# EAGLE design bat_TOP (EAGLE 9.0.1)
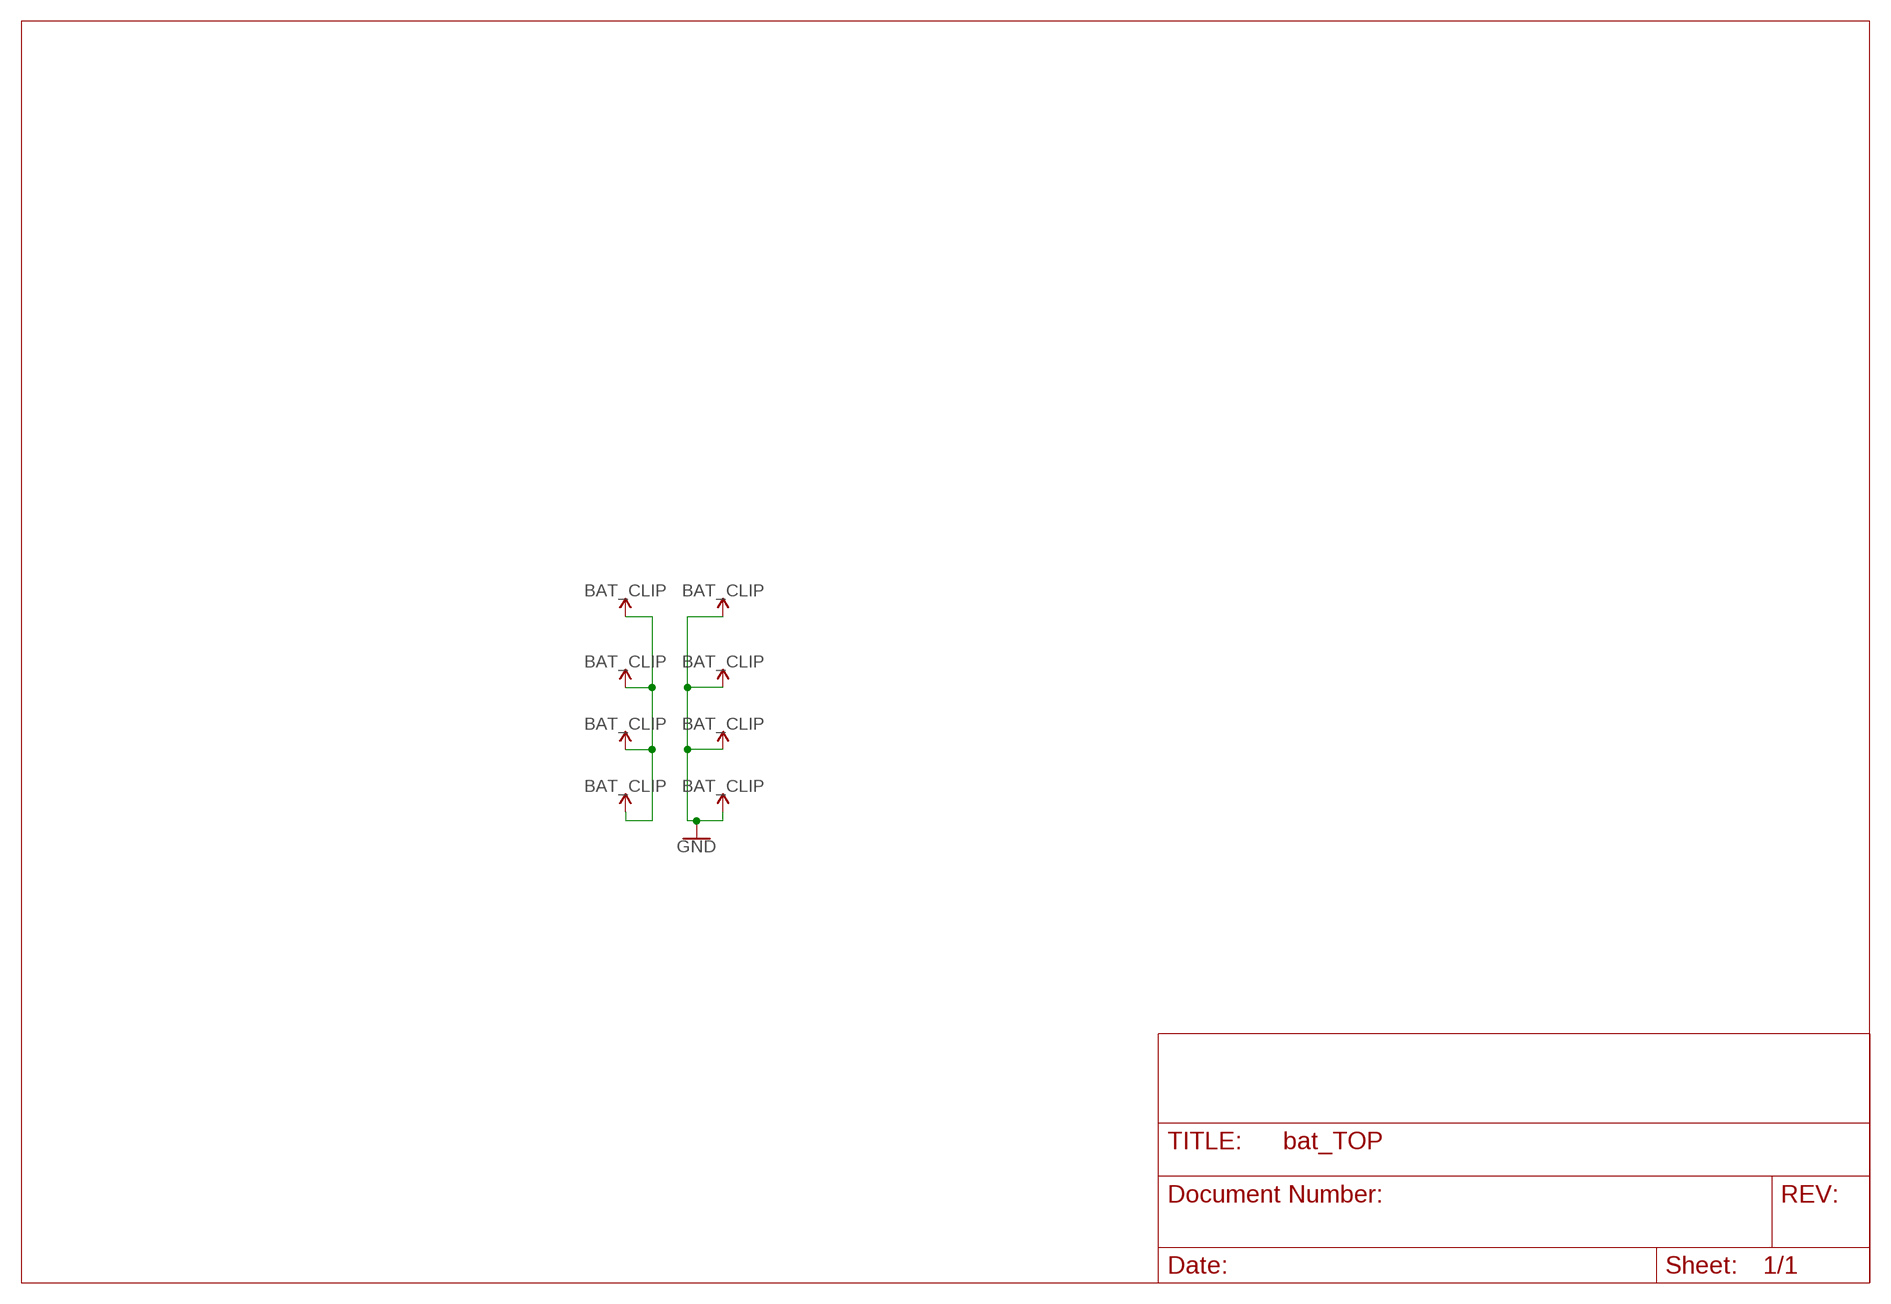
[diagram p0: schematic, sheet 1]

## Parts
U$1  BAT_CLIP  [CLIP]
U$2  BAT_CLIP  [CLIP]
U$3  BAT_CLIP  [CLIP]
U$4  BAT_CLIP  [CLIP]
U$5  BAT_CLIP  [CLIP]
U$6  BAT_CLIP  [CLIP]
U$7  BAT_CLIP  [CLIP]
U$8  BAT_CLIP  [CLIP]

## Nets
GND: U$2.P$1(V_BATT) U$2.P$2(V_BATT) U$2.P$3(V_BATT) U$2.P$4(V_BATT) U$5.P$1(V_BATT) U$5.P$2(V_BATT) U$5.P$3(V_BATT) U$5.P$4(V_BATT) U$6.P$1(V_BATT) U$6.P$2(V_BATT) U$6.P$3(V_BATT) U$6.P$4(V_BATT) U$8.P$1(V_BATT) U$8.P$2(V_BATT) U$8.P$3(V_BATT) U$8.P$4(V_BATT)
V_BATT: U$1.P$1(V_BATT) U$1.P$2(V_BATT) U$1.P$3(V_BATT) U$1.P$4(V_BATT) U$3.P$1(V_BATT) U$3.P$2(V_BATT) U$3.P$3(V_BATT) U$3.P$4(V_BATT) U$4.P$1(V_BATT) U$4.P$2(V_BATT) U$4.P$3(V_BATT) U$4.P$4(V_BATT) U$7.P$1(V_BATT) U$7.P$2(V_BATT) U$7.P$3(V_BATT) U$7.P$4(V_BATT)

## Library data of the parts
U$1-U$8 = bat:BAT_CLIP

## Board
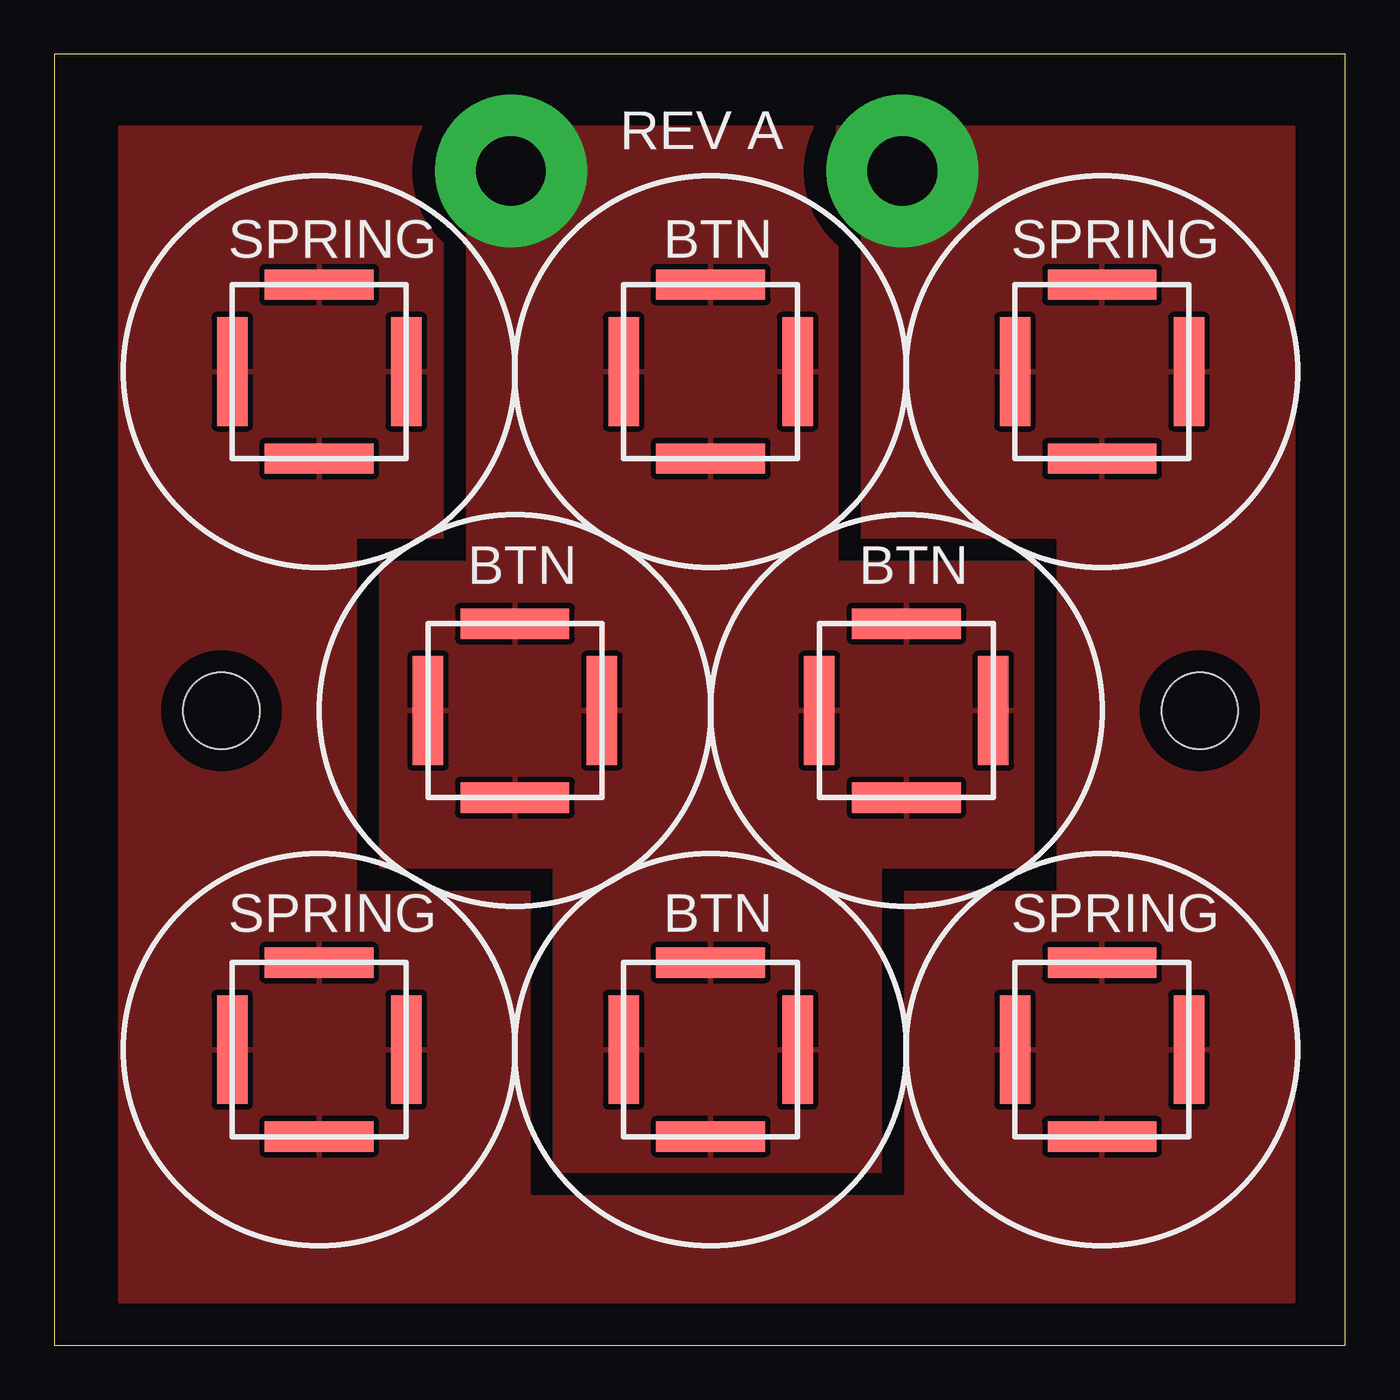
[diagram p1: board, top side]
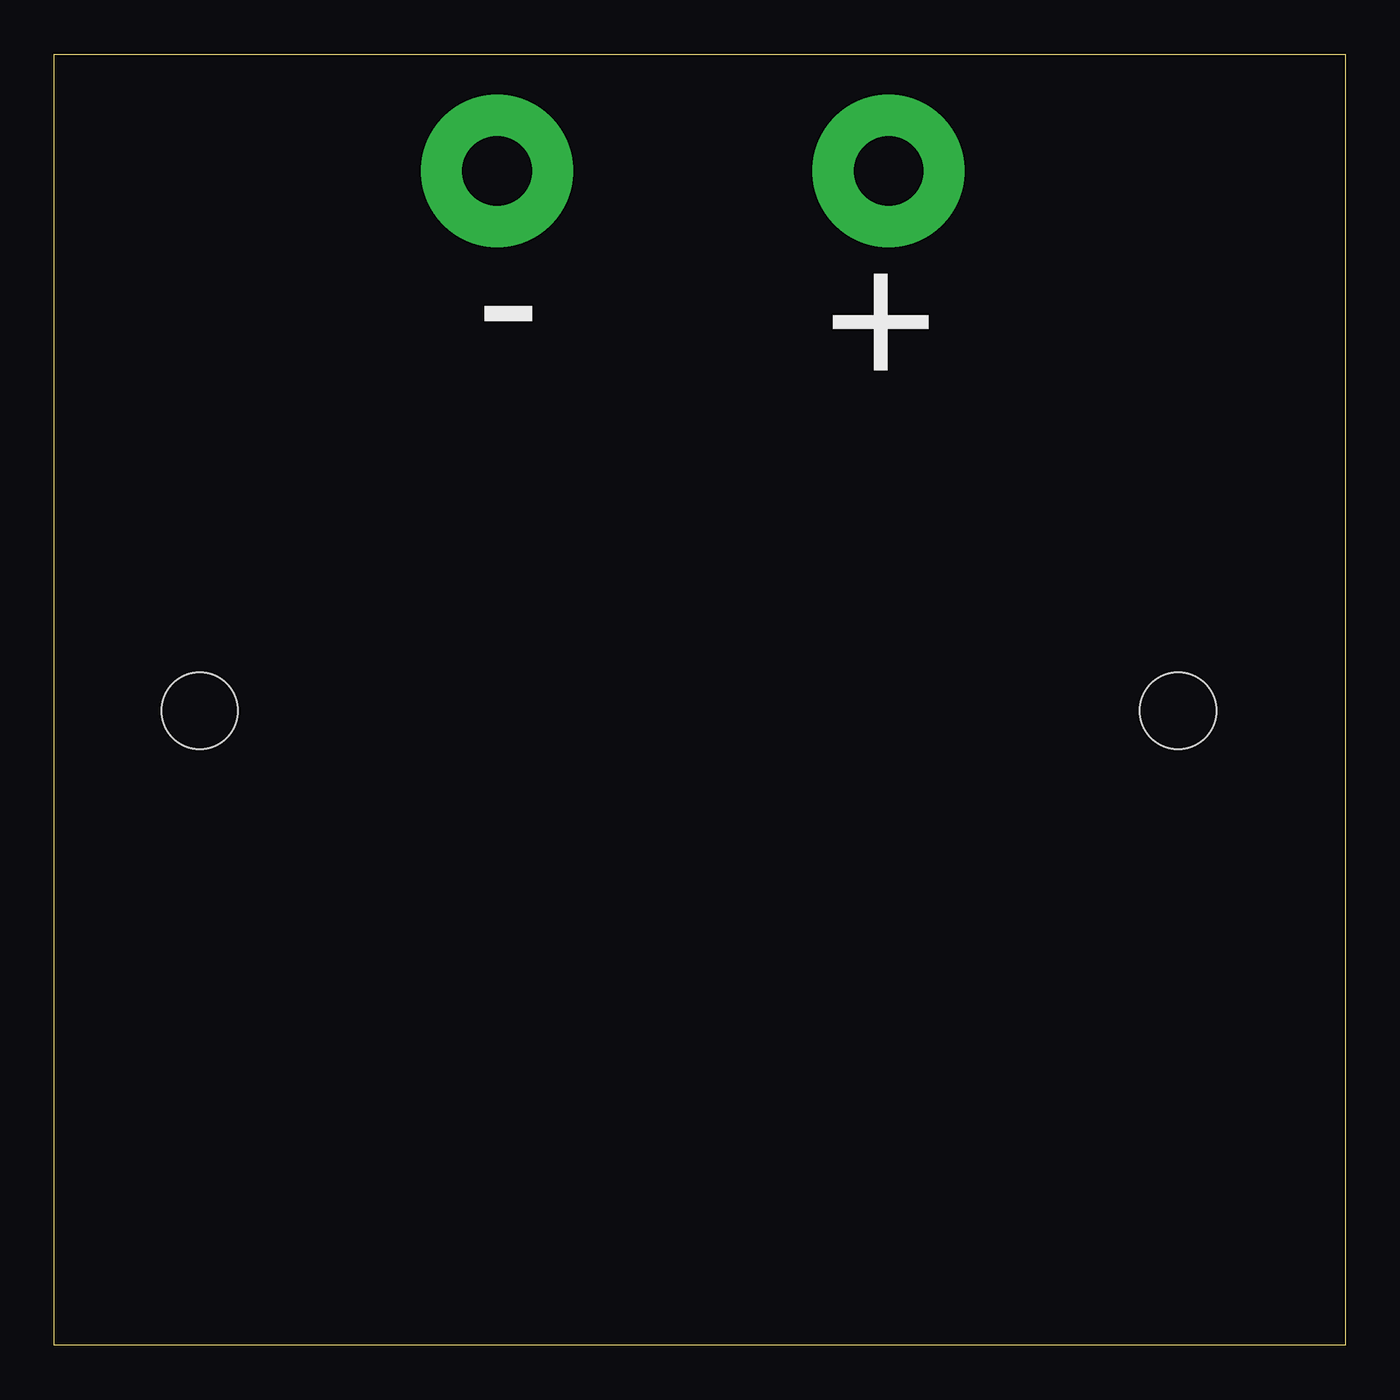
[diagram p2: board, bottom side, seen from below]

Size 59.36 x 59.36 mm. Coordinates in mm from the lower left corner, seen from the top.
Outline: 0,0 59.36,0 59.36,59.36 0,59.36 0,0
Copper layers (1*16): Top 0.035mm / dielectric 1.5mm / Bottom 0.035mm
Design rules "default": minimum track width 6mil, minimum drill 0.35mm, track to track 6mil, track to pad 6mil, pad to pad 6mil, via to via 6mil, smd to smd 6mil, copper to edge 40mil, drill to drill 6mil, minimum pad ring 10mil, minimum via ring 8mil, stop-mask expansion 4mil, vias tented up to drill 0mil, thermal gap 10mil
Holes 3.5 mm at 7.68,29.18 52.68,29.18

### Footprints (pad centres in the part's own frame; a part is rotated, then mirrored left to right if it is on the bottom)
CLIP = smd 1.4 x 5: P$1 -4,0; P$2 4,0 | smd 5 x 1.4: P$3 0,4; P$4 0,-4

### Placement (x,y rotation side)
U$1  21.18,29.18 0 top
U$2  12.18,13.59 0 top
U$3  39.18,29.18 0 top
U$4  30.18,13.59 0 top
U$5  12.18,44.77 0 top
U$6  48.18,44.77 0 top
U$7  30.18,44.77 0 top
U$8  48.18,13.59 0 top

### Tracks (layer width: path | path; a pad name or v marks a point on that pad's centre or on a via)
GND  (via drill 3.2 pad 7)
  other vias: 39,54
  pour Top (isolate 1.016, rank 2): 3,56 3,2 57,2 57,56
V_BATT  (via drill 3.2 pad 7)
  other vias: 21,54
  pour Top (isolate 1.016): 19,36 19,56 36,56 36,36 45,36 45,22 38,22 38,8 23,8 23,22 15,22 15,36

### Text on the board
tPlace: REV A | SPRING | BTN | SPRING | BTN | BTN | SPRING | BTN | SPRING
bPlace: - | +

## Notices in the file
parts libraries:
SparkFun-PowerSymbols: Licensing: Creative Commons ShareAlike 4.0 International - https://creativecommons.org/licenses/by-sa/4.0
